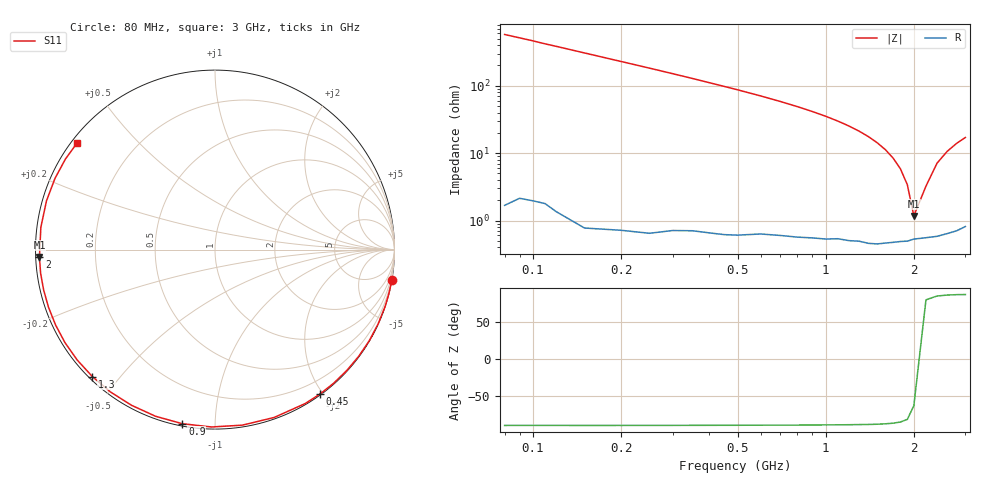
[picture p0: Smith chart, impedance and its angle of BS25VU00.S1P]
! SIEMENS Small Signal Semiconductors
! BB640
! Si Tuning Diode in SOD323
! VR = 25 V
! S-Parameters:  July  1993
# GHz  S  MA  R  50
!  f  S11
! GHz  MAG  ANG
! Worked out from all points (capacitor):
!   33 points, 80 MHz to 3 GHz, reference 50 ohm
!   read as one part to ground: C = 3.43 pF near 80 MHz
!   lowest |Z| = 1.17 ohm at 2 GHz (marker M1)
!   series resonance near 2.049 GHz, so ESL is about 1.8 nH
!   S11 on the Smith chart (normalised r, x): 80 MHz: 0, -12; 450 MHz: 0.01, -1.96; 900 MHz: 0.01, -0.83; 1.3 GHz: 0.01, -0.42; 2 GHz: 0.01, -0.02; 3 GHz: 0.02, +0.34
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0.08  0.9995 -9.9
0.15  0.9992 -18.5
0.2  0.9987 -24.6
0.25  0.9982 -30.6
0.35  0.9963 -42.5
0.4  0.9956 -48.4
0.45  0.9949 -54.1
0.5  0.994 -59.7
0.6  0.9916 -70.6
0.7  0.9899 -81.1
0.8  0.9885 -91.1
0.9  0.987 -100.6
1  0.9859 -109.6
1.1  0.9843 -118.2
1.2  0.9841 -126.3
1.3  0.9834 -134.0
1.4  0.9838 -141.3
1.5  0.9835 -148.2
1.6  0.9825 -154.7
1.7  0.9817 -160.9
1.8  0.9809 -166.7
1.9  0.9805 -172.3
2  0.979 -177.6
2.2  0.9781 172.7
2.4  0.9774 163.9
2.6  0.9758 156.0
2.8  0.9742 148.8
3  0.9712 142.3
